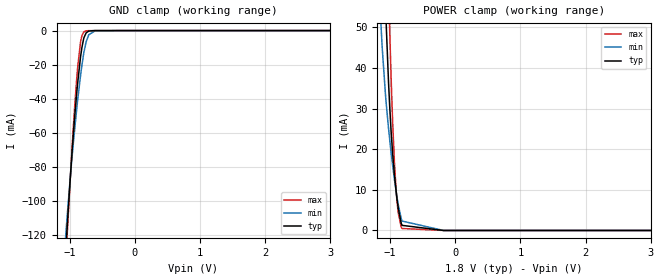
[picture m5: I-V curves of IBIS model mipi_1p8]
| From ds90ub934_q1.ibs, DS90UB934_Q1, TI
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|   mipi_1p8 Model
[Model]   mipi_1p8
Model_type   Input
Vinl = 0.63
Vinh = 1.17
|   typ   min   max
|   (nom PVT)   (fast PVT)   (slow PVT)
C_comp   3.230e-13   2.170e-13   4.390e-13
| Where nom  PVT is Nominal Process, 1.8V, 27C
|   Fast PVT is Strong Process,  1.89V, -40C
|   Slow PVT is Weak Process,   1.71V, 125C
[Voltage Range]   1.8   1.71   1.89
|Junction Temperature
[Temperature Range]   27   125   -40
[Power Clamp Reference]   1.8   1.71   1.89
[GND Clamp Reference]   0   0   0
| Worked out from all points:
|   GND clamp passes 1 mA (typ) near -0.73 V on its own axis
[GND Clamp]
|   Voltage   I(typ)   I(min)   I(max)
-1.8V     -652.8mA   -581.4mA   -709.5mA
-1.064V   -132.4mA   -122.8mA   -139.4mA
-1.044V   -119.9mA   -112.7mA   -125.2mA
-1.025V   -108.3mA   -103.4mA   -112mA
-936mV    -57.91mA   -63.62mA   -53.17mA
-877.7mV  -31.63mA   -41.62mA   -22.45mA
-828.5mV  -14.72mA   -25.59mA   -6.157mA
-777.5mV  -4.054mA   -12.37mA   -709.1uA
-744.9mV  -1.317mA   -6.537mA   -151.9uA
-703.9mV  -275.1uA   -2.396mA   -21.96uA
-608.1mV  -6.693uA   -167.6uA   -1.026uA
3.6V      0A         0A         0A
[POWER Clamp]
|   Voltage   I(typ)   I(min)   I(max)
-1.8V     575.8mA    438.5mA    682mA
-1.178V   116.2mA    62.42mA    168.3mA
-1.127V   85.15mA    46.2mA     129.9mA
-1.058V   49.75mA    30.85mA    81.31mA
-1.006V   30.21mA    22.21mA    48.7mA
-962.7mV  19.11mA    16.1mA     27.02mA
-933mV    13.44mA    12.37mA    16.24mA
-902.2mV  8.703mA    8.907mA    8.541mA
-876.6mV  5.538mA    6.396mA    4.356mA
-818.5mV  1.259mA    2.32mA     493.1uA
-180mV    2.744uA    2.358uA    3.565uA
3.6V      0A         0A         0A
